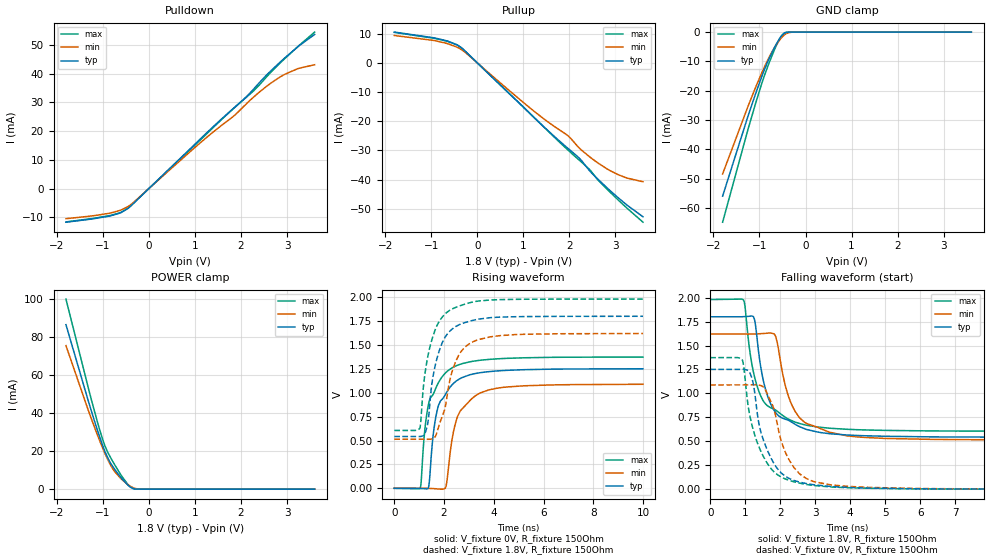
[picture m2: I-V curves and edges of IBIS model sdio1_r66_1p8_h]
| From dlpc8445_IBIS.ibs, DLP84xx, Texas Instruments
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|   r66_1p8_h
[Model]   sdio1_r66_1p8_h
Model_type   I/O
Polarity   Non-Inverting
Enable   Active-High
Vinl = 0
Vinh = 0.8
Vmeas = 0.9
Vref = 1.8
Cref = 2pF
Rref = 100000
|   typ   min   max
C_comp   4.536pF   4.091pF   4.867pF
[Voltage Range]   1.8   1.62   1.98
[Temperature Range]   27   150   -40
[Pullup Reference]   1.8   1.62   1.98
[Pulldown Reference]   0   0   0
[Power Clamp Reference]   1.8   1.62   1.98
[GND Clamp Reference]   0   0   0
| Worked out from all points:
|   slope of the pulldown table from 0 to 0.27 V, typ, clamps not added: 64.5 ohm
|   slope of the pullup table from 0 to 0.27 V, typ, clamps not added: 65.6 ohm
|   GND clamp passes 1 mA (typ) near -0.50 V on its own axis
|   POWER clamp passes 1 mA (typ) near -0.39 V on its own axis
|   falling waveform, V_fixture 1.8V, R_fixture 150Ohm: 20-80 % time 536ps typ, 606ps min, 557ps max; typ from 1.8 V to 0.542 V
|   rising waveform, V_fixture 0V, R_fixture 150Ohm: 20-80 % time 634ps typ, 692ps min, 632ps max; typ from 0 V to 1.25 V
|   rising waveform, V_fixture 1.8V, R_fixture 150Ohm: 20-80 % time 578ps typ, 701ps min, 608ps max; typ from 0.542 V to 1.8 V
|   falling waveform, V_fixture 0V, R_fixture 150Ohm: 20-80 % time 578ps typ, 624ps min, 611ps max; typ from 1.25 V to 0 V
[Pulldown]
|   Voltage   I(typ)   I(min)   I(max)
-1.8V     -11.71mA   -10.5mA    -11.62mA
-838.8mV  -9.5mA     -8.517mA   -9.364mA
-595.8mV  -8.302mA   -7.414mA   -8.207mA
-450mV    -6.897mA   -6.245mA   -6.781mA
1.364V    21.07mA    19.28mA    20.76mA
1.861V    28.31mA    25.53mA    28.2mA
2.12V     32.04mA    29.58mA    31.87mA
2.272V    34.61mA    31.85mA    34.01mA
2.542V    39.34mA    35.45mA    38.67mA
2.957V    45.61mA    39.87mA    45.37mA
3.254V    49.66mA    41.89mA    49.75mA
3.6V      53.72mA    43.15mA    54.53mA
[GND Clamp]
|   Voltage   I(typ)   I(min)   I(max)
-1.8V     -55.9mA    -48.35mA   -64.79mA
-1.244V   -28.41mA   -25.12mA   -32.87mA
-1.076V   -20.66mA   -18.55mA   -23.89mA
-952.2mV  -15.24mA   -13.97mA   -17.61mA
-806.4mV  -9.567mA   -9.046mA   -11.14mA
-633.6mV  -4.066mA   -4.277mA   -4.523mA
-552.6mV  -1.956mA   -2.515mA   -1.977mA
-504mV    -1.001mA   -1.613mA   -875.7uA
-450mV    -327.4uA   -852.5uA   -204.7uA
-358.2mV  -29.47uA   -169uA     -6.024uA
-239.4mV  -441.3nA   -11.55uA   -121.1nA
3.6V      0A         0A         0A
[Pullup]
|   Voltage   I(typ)   I(min)   I(max)
-1.8V     10.51mA    9.343mA    10.41mA
-887.4mV  8.369mA    7.468mA    8.228mA
-633.6mV  7.377mA    6.498mA    7.279mA
-352.8mV  5.249mA    4.602mA    5.246mA
1.213V    -18.42mA   -16.32mA   -18.4mA
1.964V    -29.23mA   -24.91mA   -29.79mA
2.207V    -32.54mA   -29.05mA   -33.23mA
2.434V    -36.86mA   -32.11mA   -36.44mA
2.596V    -39.49mA   -34.04mA   -39.65mA
2.839V    -43.12mA   -36.53mA   -43.61mA
3.076V    -46.44mA   -38.43mA   -47.21mA
3.6V      -52.75mA   -40.75mA   -54.6mA
[POWER Clamp]
|   Voltage   I(typ)   I(min)   I(max)
-1.8V     86.44mA    75.43mA    99.9mA
-1.244V   40.7mA     36.68mA    46.61mA
-1.082V   28.41mA    26.29mA    32.34mA
-984.6mV  21.72mA    20.5mA     24.78mA
-952.2mV  19.69mA    18.7mA     22.66mA
-855mV    14.65mA    13.73mA    17.67mA
-741.6mV  10.42mA    9.226mA    12.8mA
-595.8mV  5.783mA    5.268mA    7.056mA
-406.8mV  1.193mA    1.584mA    1.268mA
-315mV    187uA      546.2uA    116uA
-147.6mV  628.3nA    14.04uA    194.2nA
3.6V      0A         0A         0A
[Ramp]
R_load = 150
|   typ   min   max
dV/dt_r   0.750105/6.3357e-10   0.652624/7.04599e-10   0.823851/6.31648e-10
dV/dt_f   0.754398/5.35096e-10   0.663321/6.00164e-10   0.824576/5.57394e-10
[Falling Waveform]
V_fixture = 1.8V
V_fixture_min = 1.62V
V_fixture_max = 1.98V
R_fixture = 150Ohm
C_fixture = 0F
|   Time   V(typ)   V(min)   V(max)
0s        1.8V       1.619V     1.98V
955ps     1.801V     1.62V      1.975V
1.24ns    1.798V     1.62V      1.217V
1.505ns   1.158V     1.625V     929.6mV
1.83ns    820.9mV    1.62V      834.4mV
2.16ns    729.3mV    1.064V     748.3mV
2.415ns   680.8mV    820.4mV    702.4mV
2.765ns   622.6mV    684.8mV    667.3mV
3.91ns    565.9mV    557mV      625.5mV
10ns      542.5mV    513.9mV    605.6mV
[Rising Waveform]
V_fixture = 0V
V_fixture_min = 0V
V_fixture_max = 0V
R_fixture = 150Ohm
C_fixture = 0F
|   Time   V(typ)   V(min)   V(max)
0s        411.4uV    926.7uV    305.2uV
1.045ns   -1.501mV   652.4uV    2.947mV
1.225ns   -3.521mV   716.3uV    606.1mV
1.36ns    -1.362mV   -414.5uV   860mV
1.725ns   816.7mV    -5.972mV   1.08V
2.08ns    993.3mV    20.9mV     1.213V
2.38ns    1.097V     592.2mV    1.268V
2.65ns    1.148V     808.6mV    1.298V
3.805ns   1.221V     1.03V      1.349V
10ns      1.251V     1.089V     1.373V
[Rising Waveform]
V_fixture = 1.8V
V_fixture_min = 1.62V
V_fixture_max = 1.98V
R_fixture = 150Ohm
C_fixture = 0F
|   Time   V(typ)   V(min)   V(max)
0s        542.5mV    513.9mV    605.6mV
1.02ns    542.1mV    513.5mV    625.2mV
1.22ns    567.2mV    513.5mV    1.174V
1.36ns    702.9mV    513.2mV    1.395V
1.51ns    1.091V     517.4mV    1.553V
1.695ns   1.339V     569.7mV    1.69V
2.315ns   1.664V     1.213V     1.875V
2.805ns   1.731V     1.468V     1.924V
3.865ns   1.785V     1.585V     1.97V
10ns      1.8V       1.619V     1.98V
[Falling Waveform]
|Gnd
V_fixture = 0V
V_fixture_min = 0V
V_fixture_max = 0V
R_fixture = 150Ohm
C_fixture = 0F
|   Time   V(typ)   V(min)   V(max)
0s        1.251V     1.089V     1.373V
910ps     1.251V     1.089V     1.355V
1.115ns   1.227V     1.089V     801.3mV
1.23ns    1.104V     1.089V     620.7mV
1.535ns   499.9mV    1.061V     331.8mV
1.81ns    276.7mV    849.3mV    186.6mV
2.21ns    121.3mV    337.6mV    98.03mV
2.745ns   59.04mV    112.1mV    49.75mV
3.425ns   28.89mV    46.54mV    24.03mV
10ns      411.4uV    926.9uV    305.2uV
